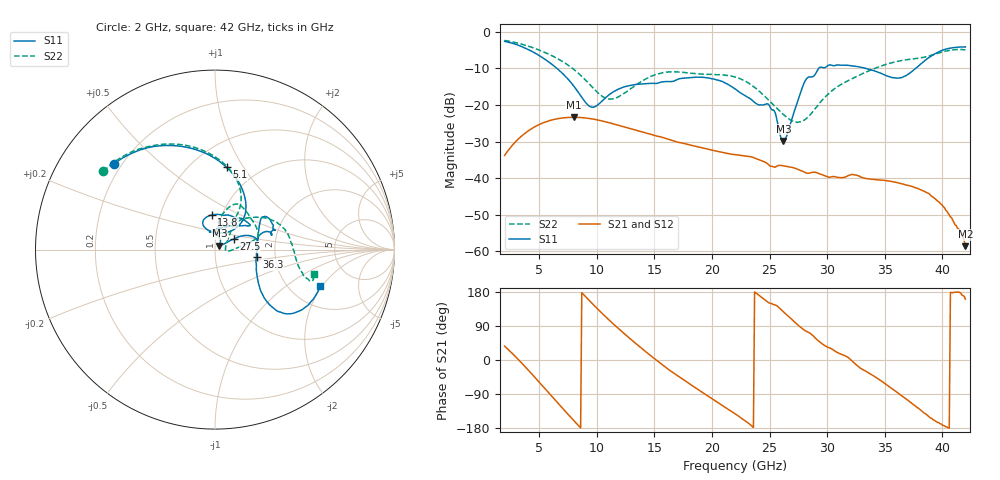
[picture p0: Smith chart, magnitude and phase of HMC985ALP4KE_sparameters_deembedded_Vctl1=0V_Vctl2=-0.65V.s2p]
!s2p File: Measurements: S11, S21, S12, S22
# GHz S dB R 50.0
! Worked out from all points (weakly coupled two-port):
!   401 points, 2 GHz to 42 GHz, reference 50 ohm
!   highest |S21| = -23.36 dB at 8 GHz (marker M1); lowest = -58.6 dB at 42 GHz (marker M2)
!   lowest |S11| = -29.8 dB at 26.2 GHz (marker M3), VSWR 1.07, Z = 52.4 + j2.24 ohm
!   |S11| at or under -10 dB: 6.539 GHz to 29.27 GHz (22.74 GHz wide, 127 % of centre); 33.34 GHz to 37.69 GHz (4.346 GHz wide, 12.2 % of centre)
!   |S22| runs from -24.8 to -2.4 dB; largest |S21 - S12| = 0.00015
!   S11 on the Smith chart (normalised r, x): 2 GHz: 0.17, +0.36; 5.1 GHz: 0.73, +0.85; 13.8 GHz: 0.90, +0.36; 27.5 GHz: 1.22, +0.15; 36.3 GHz: 1.59, -0.14; 42 GHz: 2.91, -1.91
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2  -2.62 139.8  -33.78 36.6  -33.78 36.6  -2.38 145.0
3.5  -4.09 112.0  -28.42 -8.6  -28.43 -8.6  -3.41 120.9
5.1  -6.70 81.9  -25.20 -61.7  -25.20 -61.7  -5.13 96.5
8  -14.82 45.3  -23.36 -159.7  -23.36 -159.7  -10.26 61.8
8.7  -17.93 51.7  -23.45 177.6  -23.45 177.6  -12.19 58.1
9.7  -20.61 86.4  -23.86 146.1  -23.86 146.1  -15.42 59.1
11.1  -17.14 115.3  -24.86 104.6  -24.87 104.6  -18.39 74.6
13.8  -14.27 95.2  -27.21 33.1  -27.21 33.1  -13.71 77.3
15.4  -13.94 73.0  -28.61 -5.3  -28.61 -5.3  -11.42 68.3
19.4  -12.52 34.7  -31.91 -90.2  -31.92 -90.1  -11.61 35.3
22  -15.59 52.3  -33.55 -141.8  -33.56 -141.8  -12.36 15.6
25  -20.21 97.7  -36.54 150.1  -36.55 150.1  -18.95 2.5
26.2  -29.82 41.3  -36.62 126.9  -36.62 127.0  -22.60 -6.5
27.5  -18.41 29.7  -37.66 91.3  -37.64 91.2  -24.68 2.8
28.1  -13.37 20.7  -38.43 77.1  -38.43 77.2  -23.95 18.1
28.7  -12.31 12.8  -38.40 65.9  -38.42 66.0  -22.02 31.9
31  -9.09 23.4  -39.80 18.1  -39.84 18.3  -14.78 51.9
33.3  -9.96 34.5  -40.04 -28.4  -40.03 -28.4  -11.14 40.3
35.4  -12.27 12.4  -40.79 -70.9  -40.79 -70.8  -8.65 24.9
36.3  -12.58 -10.2  -41.33 -90.8  -41.39 -90.8  -7.97 17.4
39.8  -5.31 -41.3  -46.82 -168.0  -46.75 -168.1  -5.67 -16.4
42  -4.14 -19.0  -58.55 160.6  -58.78 161.5  -4.95 -14.0
